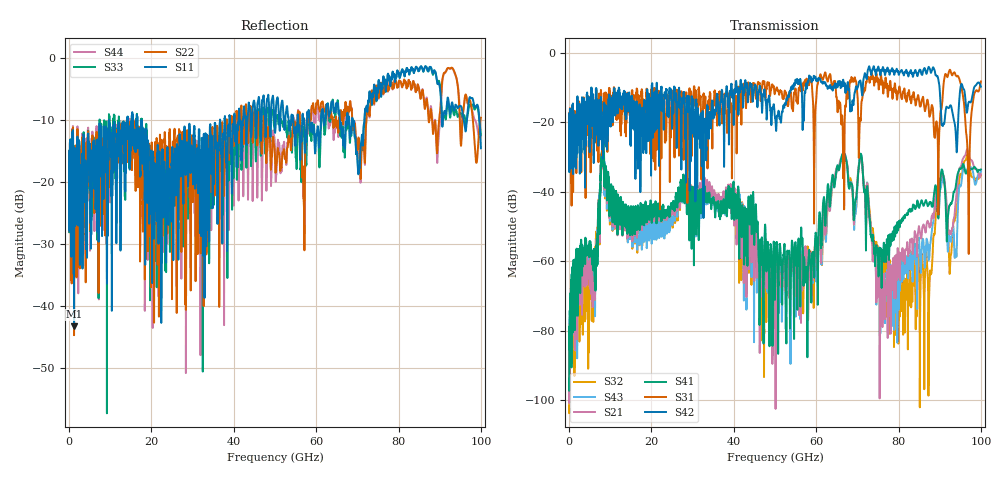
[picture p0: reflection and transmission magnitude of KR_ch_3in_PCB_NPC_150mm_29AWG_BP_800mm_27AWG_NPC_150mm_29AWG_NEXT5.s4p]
# GHz S RI R 45
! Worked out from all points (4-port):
!   4000 points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, 25 MHz to 100 GHz, reference 45 ohm
!   strongest paths, dB at 25 MHz, 25.02 GHz, 50.02 GHz, 75.03 GHz, 100 GHz:
!     S42: -22.2, -20.8, -18.7, -4.1, -9.8
!     S31: -22.2, -12.0, -11.5, -7.8, -8.3
!     S41: -93.8, -44.1, -69.3, -59.3, -33.6
!     S21: -97.5, -45.1, -62.2, -62.0, -35.0
!     S43: -96.3, -48.4, -65.5, -61.8, -34.1
!     S32: -101.7, -48.4, -69.9, -58.0, -35.3
!   lowest |S11| = -43.2 dB at 1.225 GHz (marker M1), VSWR 1.01, Z = 44.9 - j0.618 ohm
!   |S11| at or under -10 dB: start of sweep to 14.14 GHz; 16.58 GHz to 36.66 GHz (20.08 GHz wide, 75.4 % of centre); 68.84 GHz to 71.74 GHz (2.898 GHz wide, 4.12 % of centre)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
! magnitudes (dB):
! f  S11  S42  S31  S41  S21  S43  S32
! 25 MHz  -17.4  -22.2  -22.2  -93.8  -97.5  -96.3  -101.7
! 1.225 GHz  -43.2  -25.9  -25.3  -66.4  -71.8  -70.5  -83.0
! 8.125 GHz  -15.2  -21.3  -26.6  -28.4  -29.0  -28.2  -28.9
! 49.8 GHz  -9.1  -15.6  -10.6  -55.3  -56.5  -70.6  -61.6
! 70.8 GHz  -14.4  -8.3  -19.5  -29.1  -29.9  -29.0  -29.6
! 75.85 GHz  -5.5  -4.9  -7.4  -62.2  -61.7  -60.4  -60.0
! 100 GHz  -14.6  -9.8  -8.3  -33.6  -35.0  -34.1  -35.3
